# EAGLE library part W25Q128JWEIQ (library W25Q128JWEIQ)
NOR Flash spiFlash, 128M-bit, 4Kb Uniform Sector Source: Datasheet
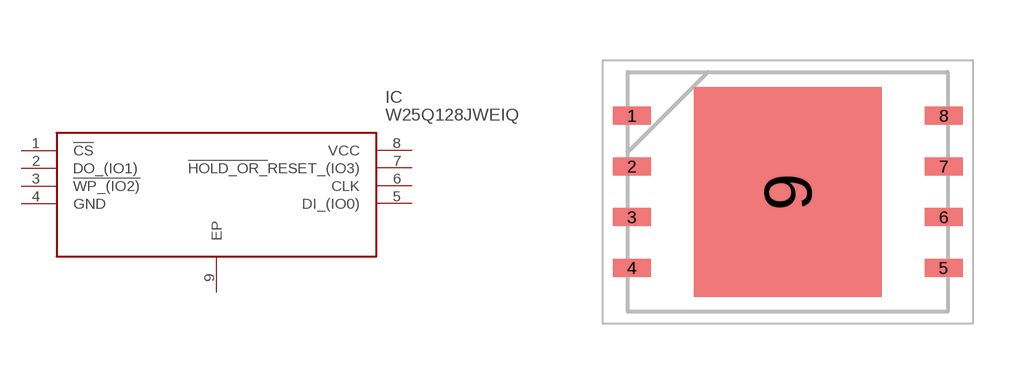
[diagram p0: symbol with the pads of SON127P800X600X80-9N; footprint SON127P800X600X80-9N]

Designator prefix IC

## W25Q128JWEIQ (Arrow_Part_Number: W25Q128JWEIQ; Arrow_Price-Stock: https://www.arrow.com/en/products/w25q128jweiq/winbond-electronics?region=nac; Description: NOR Flash spiFlash, 128M-bit, 4Kb Uniform Sector; Height: 0.8mm; Manufacturer_Name: Winbond; Manufacturer_Part_Number: W25Q128JWEIQ; Mouser_Part_Number: 454-W25Q128JWEIQ; Mouser_Price-Stock: https://www.mouser.co.uk/ProductDetail/Winbond/W25Q128JWEIQ?qs=PqoDHHvF64%252B7VGysTrW%2FEA%3D%3D)  [SON127P800X600X80-9N]
1  !CS
2  DO_(IO1)
3  !WP_(IO2)
4  GND
5  DI_(IO0)
6  CLK
7  !HOLD_OR_!RESET_(IO3)
8  VCC
9  EP

## Footprint SON127P800X600X80-9N (pad centres in mm)
WSON-8 8x6-mm_
smd 0.95 x 0.45: 1 -3.9,1.905; 2 -3.9,0.635; 3 -3.9,-0.635; 4 -3.9,-1.905; 5 3.9,-1.905; 6 3.9,-0.635; 7 3.9,0.635; 8 3.9,1.905
smd 4.7 x 5.25: 9 0,0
